| TEXAS INSTRUMENTS INCORPORATED
| Standard Linear and Logic Group
| IBIS Model of SN74LVCH245A
| OCTAL BUS TRANSCEIVERS WITH 3-STATE OUTPUTS
| This file contains package information for the following:
|  TSSOP 20-pin (PW) package as [Component] LVCH245A_PW
|  SOP 20-pin (NS) package as [Component] LVCH245A_NS
|  SOIC 20-pin (DW) package as [Component] LVCH245A_DW
|  TVSOP 20-pin (DGV) package as [Component] LVCH245A_DGV
|  SSOP 20-pin (DB) package as [Component] LVCH245A_DB
|  QFN 20-pin (RGY) package as [Component] LVCH245A_RGY
|  VFBGA 20-pin (GQN) package as [Component] LVCH245A_GQN
|  VFBGA 20-pin (ZQN) package as [Component] LVCH245A_ZQN
| This device can be powered at the following Vccs:
|  1.8 volt Vcc
|  2.5 volt Vcc
|  3.3 volt Vcc
| This file provides unique models under the [Model Selector] for each Vcc.
| For operation at a specific Vcc, select the appropriate model after each
| [Model Selector] keyword.
[IBIS Ver]   3.2
[Comment char]  |_char
[File Name]   sn74lvch245a.ibs
[File Rev]   1.2 | e_die
[Date]   November 10, 2005
[Source]   Data created from TI-SPICE simulations at TI-SLL.
[Notes]   The following is an IBIS list for the LVCH245A.
   Please contact sllibis@ti.com with questions and
   comments concerning SLL IBIS models.
   - FILE REV HISTORY
   - 1.1 Release IBIS file on 4/25/02
   - 1.2 RGY and ZQN pacakages added 11/10/05
   - Non-monotonic data in ground-clamp due to bus-hold
   - Due to the fact that the device is 5-V input/output
   tolerant, the output model has some Non-monotonic
   warnings.
[Disclaimer] Property of Texas Instruments Incorporated.  Unauthorized
   reproduction and/or distribution is strictly prohibited.
   This product is protected under copyright law.
   Created  2002, (C) Copyright  2002, Texas Instruments
   Incorporated, All Rights Reserved
   UNLESS THERE IS A SIGNED, WRITTEN AGREEMENT TO THE
   CONTRARY, TEXAS INSTRUMENTS (TI) IS PROVIDING THE IBIS
   MODELS  AND WITHOUT ANY WARRANTY, EXPRESSED OR
   IMPLIED.  TI assumes no liability for:
   1) the accuracy of the IBIS models provided to your
   company;
   2) the proper functioning of these IBIS Models in your
   design or for any resulting applications; or
   3) infringement of patents, copyrights or intellectual
   property rights resulting from your use of these IBIS
   models.
   TI provides IBIS Models as a service to our customers.
   You and your company shall not distribute, sell or give
   these models to anyone else without prior written
   permission from TI.
   TI reserves the right to make changes to our products or
   to discontinue any semiconductor product or service
   without notice, and advises our customers to obtain the
   latest version of relevant information to verify, before
   placing orders, that the information being relied on is
   current.
   Please be aware that your receipt and use of the IBIS
   information provided shall serve as acceptance of these
   terms and conditions.  If you do not accept these terms,
   you should return or destroy the IBIS models and any
   other accompanying information immediately.
| Component LVCH245A_PW 20-pin TSSOP
[Component]   LVCH245A_PW
[Manufacturer]   Texas Instruments, Inc.
[Package]
|   typ   min   max
R_pkg   4.500e-02   3.600e-02   5.700e-02
L_pkg   2.694e-09   2.290e-09   3.177e-09
C_pkg   1.560e-13   7.600e-14   2.590e-13
[Pin]   signal_name   model_name   R_pin   L_pin   C_pin
1   DIR   LVCH245A_IN   3.600e-02   3.045e-09   2.590e-13
2   A1   LVCH245A_IO   5.100e-02   3.013e-09   1.890e-13
3   A2   LVCH245A_IO   4.400e-02   2.695e-09   1.640e-13
4   A3   LVCH245A_IO   4.700e-02   2.362e-09   7.900e-14
5   A4   LVCH245A_IO   4.700e-02   2.333e-09   8.600e-14
6   A5   LVCH245A_IO   4.700e-02   2.298e-09   8.500e-14
7   A6   LVCH245A_IO   4.700e-02   2.351e-09   7.900e-14
8   A7   LVCH245A_IO   4.400e-02   2.706e-09   1.650e-13
9   A8   LVCH245A_IO   4.900e-02   2.999e-09   1.880e-13
10   GND   GND   3.900e-02   3.039e-09   2.570e-13
11   B8   LVCH245A_IO   3.800e-02   3.044e-09   2.580e-13
12   B7   LVCH245A_IO   5.700e-02   3.177e-09   1.990e-13
13   B6   LVCH245A_IO   4.400e-02   2.825e-09   1.730e-13
14   B5   LVCH245A_IO   4.700e-02   2.429e-09   8.300e-14
15   B4   LVCH245A_IO   4.900e-02   2.383e-09   9.000e-14
16   B3   LVCH245A_IO   4.900e-02   2.347e-09   8.900e-14
17   B2   LVCH245A_IO   4.700e-02   2.290e-09   7.600e-14
18   B1   LVCH245A_IO   4.500e-02   2.613e-09   1.580e-13
19   NOE   LVCH245A_IN   4.400e-02   2.883e-09   1.810e-13
20   VCC   POWER   3.900e-02   3.044e-09   2.560e-13
| Component LVCH245A_NS 20-pin SOP
[Component]   LVCH245A_NS
[Manufacturer]   Texas Instruments, Inc.
[Package]
|   typ   min   max
R_pkg   4.400e-02   2.900e-02   5.800e-02
L_pkg   3.666e-09   2.317e-09   5.115e-09
C_pkg   5.480e-13   3.160e-13   7.250e-13
[Pin]   signal_name   model_name   R_pin   L_pin   C_pin
1   DIR   LVCH245A_IN   5.800e-02   5.115e-09   7.250e-13
2   A1   LVCH245A_IO   5.300e-02   4.591e-09   7.240e-13
3   A2   LVCH245A_IO   4.900e-02   3.754e-09   5.720e-13
4   A3   LVCH245A_IO   2.900e-02   2.549e-09   3.880e-13
5   A4   LVCH245A_IO   3.100e-02   2.317e-09   3.160e-13
6   A5   LVCH245A_IO   3.100e-02   2.317e-09   3.160e-13
7   A6   LVCH245A_IO   2.900e-02   2.556e-09   3.990e-13
8   A7   LVCH245A_IO   4.900e-02   3.754e-09   5.790e-13
9   A8   LVCH245A_IO   5.300e-02   4.591e-09   7.240e-13
10   GND   GND   5.800e-02   5.115e-09   7.250e-13
11   B8   LVCH245A_IO   5.800e-02   5.115e-09   7.250e-13
12   B7   LVCH245A_IO   5.300e-02   4.591e-09   7.240e-13
13   B6   LVCH245A_IO   4.900e-02   3.754e-09   5.790e-13
14   B5   LVCH245A_IO   2.900e-02   2.557e-09   3.990e-13
15   B4   LVCH245A_IO   3.100e-02   2.317e-09   3.160e-13
16   B3   LVCH245A_IO   3.100e-02   2.317e-09   3.160e-13
17   B2   LVCH245A_IO   2.900e-02   2.557e-09   3.990e-13
18   B1   LVCH245A_IO   4.900e-02   3.754e-09   5.790e-13
19   NOE   LVCH245A_IN   5.300e-02   4.591e-09   7.240e-13
20   VCC   POWER   5.800e-02   5.115e-09   7.250e-13
| Component LVCH245A_DW 20-pin SOIC
[Component]   LVCH245A_DW
[Manufacturer]   Texas Instruments, Inc.
[Package]
|   typ   min   max
R_pkg   3.800e-02   3.300e-02   4.500e-02
L_pkg   5.012e-09   4.110e-09   6.349e-09
C_pkg   7.170e-13   5.300e-13   8.680e-13
[Pin]   signal_name   model_name   R_pin   L_pin   C_pin
1   DIR   LVCH245A_IN   4.200e-02   6.336e-09   8.650e-13
2   A1   LVCH245A_IO   4.300e-02   5.542e-09   8.670e-13
3   A2   LVCH245A_IO   3.400e-02   4.714e-09   7.320e-13
4   A3   LVCH245A_IO   3.400e-02   4.377e-09   5.910e-13
5   A4   LVCH245A_IO   3.600e-02   4.130e-09   5.330e-13
6   A5   LVCH245A_IO   3.500e-02   4.111e-09   5.300e-13
7   A6   LVCH245A_IO   3.400e-02   4.284e-09   5.830e-13
8   A7   LVCH245A_IO   3.400e-02   4.634e-09   7.260e-13
9   A8   LVCH245A_IO   4.000e-02   5.518e-09   8.650e-13
10   GND   GND   4.300e-02   6.349e-09   8.660e-13
11   B8   LVCH245A_IO   4.100e-02   6.281e-09   8.610e-13
12   B7   LVCH245A_IO   4.500e-02   5.561e-09   8.680e-13
13   B6   LVCH245A_IO   3.300e-02   4.778e-09   7.420e-13
14   B5   LVCH245A_IO   3.500e-02   4.414e-09   5.960e-13
15   B4   LVCH245A_IO   3.500e-02   4.110e-09   5.330e-13
16   B3   LVCH245A_IO   3.600e-02   4.130e-09   5.330e-13
17   B2   LVCH245A_IO   3.400e-02   4.377e-09   5.910e-13
18   B1   LVCH245A_IO   3.400e-02   4.714e-09   7.310e-13
19   NOE   LVCH245A_IN   4.300e-02   5.569e-09   8.680e-13
20   VCC   POWER   4.200e-02   6.308e-09   8.640e-13
| Component LVCH245A_DGV 20-pin TVSOP
[Component]   LVCH245A_DGV
[Manufacturer]   Texas Instruments, Inc.
[Package]
|   typ   min   max
R_pkg   4.400e-02   3.800e-02   4.800e-02
L_pkg   2.561e-09   2.236e-09   2.961e-09
C_pkg   3.420e-13   2.640e-13   4.460e-13
[Pin]   signal_name   model_name   R_pin   L_pin   C_pin
1   DIR   LVCH245A_IN   4.400e-02   2.935e-09   4.170e-13
2   A1   LVCH245A_IO   4.200e-02   2.869e-09   4.460e-13
3   A2   LVCH245A_IO   4.300e-02   2.399e-09   3.160e-13
4   A3   LVCH245A_IO   4.400e-02   2.236e-09   2.650e-13
5   A4   LVCH245A_IO   4.600e-02   2.278e-09   2.640e-13
6   A5   LVCH245A_IO   4.500e-02   2.274e-09   2.640e-13
7   A6   LVCH245A_IO   4.400e-02   2.285e-09   2.690e-13
8   A7   LVCH245A_IO   4.300e-02   2.452e-09   3.200e-13
9   A8   LVCH245A_IO   4.400e-02   2.900e-09   4.460e-13
10   GND   GND   4.400e-02   2.961e-09   4.180e-13
11   B8   LVCH245A_IO   4.500e-02   2.954e-09   4.180e-13
12   B7   LVCH245A_IO   4.200e-02   2.847e-09   4.430e-13
13   B6   LVCH245A_IO   4.500e-02   2.453e-09   3.190e-13
14   B5   LVCH245A_IO   4.500e-02   2.297e-09   2.690e-13
15   B4   LVCH245A_IO   4.800e-02   2.334e-09   2.680e-13
16   B3   LVCH245A_IO   4.800e-02   2.335e-09   2.670e-13
17   B2   LVCH245A_IO   4.600e-02   2.299e-09   2.680e-13
18   B1   LVCH245A_IO   4.600e-02   2.457e-09   3.200e-13
19   NOE   LVCH245A_IN   4.300e-02   2.848e-09   4.410e-13
20   VCC   POWER   3.800e-02   2.812e-09   4.080e-13
| Component LVCH245A_DB 20-pin SSOP
[Component]   LVCH245A_DB
[Manufacturer]   Texas Instruments, Inc.
[Package]
|   typ   min   max
R_pkg   4.000e-02   3.500e-02   5.100e-02
L_pkg   3.495e-09   3.035e-09   4.314e-09
C_pkg   4.200e-13   3.460e-13   5.020e-13
[Pin]   signal_name   model_name   R_pin   L_pin   C_pin
1   DIR   LVCH245A_IN   4.900e-02   4.310e-09   5.020e-13
2   A1   LVCH245A_IO   4.800e-02   3.903e-09   4.870e-13
3   A2   LVCH245A_IO   3.500e-02   3.189e-09   3.960e-13
4   A3   LVCH245A_IO   3.500e-02   3.036e-09   3.470e-13
5   A4   LVCH245A_IO   3.500e-02   3.035e-09   3.670e-13
6   A5   LVCH245A_IO   3.500e-02   3.035e-09   3.670e-13
7   A6   LVCH245A_IO   3.500e-02   3.036e-09   3.470e-13
8   A7   LVCH245A_IO   3.500e-02   3.189e-09   3.970e-13
9   A8   LVCH245A_IO   4.700e-02   3.899e-09   4.880e-13
10   GND   GND   5.100e-02   4.314e-09   5.000e-13
11   B8   LVCH245A_IO   5.100e-02   4.314e-09   5.000e-13
12   B7   LVCH245A_IO   4.700e-02   3.899e-09   4.880e-13
13   B6   LVCH245A_IO   3.500e-02   3.189e-09   3.970e-13
14   B5   LVCH245A_IO   3.500e-02   3.036e-09   3.460e-13
15   B4   LVCH245A_IO   3.500e-02   3.035e-09   3.670e-13
16   B3   LVCH245A_IO   3.500e-02   3.035e-09   3.670e-13
17   B2   LVCH245A_IO   3.500e-02   3.036e-09   3.460e-13
18   B1   LVCH245A_IO   3.500e-02   3.189e-09   3.970e-13
19   NOE   LVCH245A_IN   4.700e-02   3.899e-09   4.880e-13
20   VCC   POWER   5.100e-02   4.314e-09   5.020e-13
| Component LVCH245A_RGY 20-pin QFN
[Component]   LVCH245A_RGY
[Manufacturer]   Texas Instruments, Inc.
[Package]
|   typ   min   max
R_pkg   5.000e-02   4.600e-02   5.500e-02
L_pkg   1.119e-09   1.025e-09   1.227e-09
C_pkg   3.520e-13   3.440e-13   3.630e-13
[Pin]   signal_name   model_name   R_pin   L_pin   C_pin
1   DIR   LVCH245A_IN   5.200e-02   1.167e-09   3.600e-13
2   A1   LVCH245A_IO   4.700e-02   1.049e-09   3.440e-13
3   A2   LVCH245A_IO   4.700e-02   1.055e-09   3.450e-13
4   A3   LVCH245A_IO   5.000e-02   1.119e-09   3.500e-13
5   A4   LVCH245A_IO   5.500e-02   1.227e-09   3.600e-13
6   A5   LVCH245A_IO   5.200e-02   1.167e-09   3.550e-13
7   A6   LVCH245A_IO   4.900e-02   1.087e-09   3.480e-13
8   A7   LVCH245A_IO   4.700e-02   1.054e-09   3.460e-13
9   A8   LVCH245A_IO   4.900e-02   1.091e-09   3.490e-13
10   GND   GND   5.300e-02   1.184e-09   3.620e-13
11   B8   LVCH245A_IO   5.300e-02   1.181e-09   3.600e-13
12   B7   LVCH245A_IO   5.000e-02   1.108e-09   3.490e-13
13   B6   LVCH245A_IO   4.800e-02   1.075e-09   3.470e-13
14   B5   LVCH245A_IO   5.000e-02   1.107e-09   3.490e-13
15   B4   LVCH245A_IO   5.400e-02   1.200e-09   3.620e-13
16   B3   LVCH245A_IO   5.100e-02   1.141e-09   3.570e-13
17   B2   LVCH245A_IO   4.700e-02   1.043e-09   3.440e-13
18   B1   LVCH245A_IO   4.600e-02   1.025e-09   3.440e-13
19   NOE   LVCH245A_IN   4.900e-02   1.090e-09   3.490e-13
20   VCC   POWER   5.400e-02   1.204e-09   3.630e-13
| Component LVCH245A_GQN 20-pin VFBGA
[Component]   LVCH245A_GQN
[Manufacturer] Texas Instruments, Inc.
[Package]
|   typ   min   max
R_pkg   4.300e-02   3.300e-02   6.100e-02
L_pkg   1.317e-09   8.960e-10   2.088e-09
C_pkg   1.130e-13   6.400e-14   1.900e-13
[Pin]   signal_name   model_name   R_pin   L_pin   C_pin
A2   DIR   LVCH245A_IN   3.800e-02   1.199e-09   1.210e-13
A1   A1   LVCH245A_IO   4.000e-02   1.067e-09   1.020e-13
B3   A2   LVCH245A_IO   6.100e-02   1.999e-09   1.900e-13
B1   A3   LVCH245A_IO   3.300e-02   9.630e-10   7.100e-14
C2   A4   LVCH245A_IO   4.900e-02   1.523e-09   1.230e-13
C1   A5   LVCH245A_IO   3.300e-02   8.960e-10   6.400e-14
D3   A6   LVCH245A_IO   6.100e-02   1.899e-09   1.640e-13
D1   A7   LVCH245A_IO   3.300e-02   8.980e-10   6.700e-14
E2   A8   LVCH245A_IO   4.900e-02   1.514e-09   1.280e-13
E1   GND   GND   3.600e-02   1.006e-09   9.400e-14
E3   B8   LVCH245A_IO   4.900e-02   1.683e-09   1.460e-13
E4   B7   LVCH245A_IO   3.300e-02   1.121e-09   8.900e-14
D2   B6   LVCH245A_IO   6.100e-02   2.088e-09   1.730e-13
D4   B5   LVCH245A_IO   3.300e-02   1.027e-09   7.100e-14
C3   B4   LVCH245A_IO   4.900e-02   1.558e-09   1.240e-13
C4   B3   LVCH245A_IO   3.300e-02   9.280e-10   6.700e-14
B2   B2   LVCH245A_IO   6.100e-02   1.921e-09   1.770e-13
B4   B1   LVCH245A_IO   3.300e-02   9.010e-10   7.700e-14
A4   NOE   LVCH245A_IN   3.700e-02   9.900e-10   9.800e-14
A3   VCC   POWER   3.500e-02   1.168e-09   1.190e-13
| Component LVCH245A_ZQN 20-pin VFBGA
[Component]   LVCH245A_ZQN
[Manufacturer] Texas Instruments, Inc.
[Package]
|   typ   min   max
R_pkg   4.300e-02   3.300e-02   6.100e-02
L_pkg   1.317e-09   8.960e-10   2.088e-09
C_pkg   1.130e-13   6.400e-14   1.900e-13
[Pin]   signal_name   model_name   R_pin   L_pin   C_pin
A2   DIR   LVCH245A_IN   3.800e-02   1.199e-09   1.210e-13
A1   A1   LVCH245A_IO   4.000e-02   1.067e-09   1.020e-13
B3   A2   LVCH245A_IO   6.100e-02   1.999e-09   1.900e-13
B1   A3   LVCH245A_IO   3.300e-02   9.630e-10   7.100e-14
C2   A4   LVCH245A_IO   4.900e-02   1.523e-09   1.230e-13
C1   A5   LVCH245A_IO   3.300e-02   8.960e-10   6.400e-14
D3   A6   LVCH245A_IO   6.100e-02   1.899e-09   1.640e-13
D1   A7   LVCH245A_IO   3.300e-02   8.980e-10   6.700e-14
E2   A8   LVCH245A_IO   4.900e-02   1.514e-09   1.280e-13
E1   GND   GND   3.600e-02   1.006e-09   9.400e-14
E3   B8   LVCH245A_IO   4.900e-02   1.683e-09   1.460e-13
E4   B7   LVCH245A_IO   3.300e-02   1.121e-09   8.900e-14
D2   B6   LVCH245A_IO   6.100e-02   2.088e-09   1.730e-13
D4   B5   LVCH245A_IO   3.300e-02   1.027e-09   7.100e-14
C3   B4   LVCH245A_IO   4.900e-02   1.558e-09   1.240e-13
C4   B3   LVCH245A_IO   3.300e-02   9.280e-10   6.700e-14
B2   B2   LVCH245A_IO   6.100e-02   1.921e-09   1.770e-13
B4   B1   LVCH245A_IO   3.300e-02   9.010e-10   7.700e-14
A4   NOE   LVCH245A_IN   3.700e-02   9.900e-10   9.800e-14
A3   VCC   POWER   3.500e-02   1.168e-09   1.190e-13
| Model LVCH245A_IN
[Model Selector]   LVCH245A_IN
LVCH245A_IN_18   1.8 volt Vcc
LVCH245A_IN_25   2.5 volt Vcc
LVCH245A_IN_33   3.3 volt Vcc
| Model LVCH245A_IO
[Model Selector]   LVCH245A_IO
LVCH245A_IO_18   1.8 volt Vcc
LVCH245A_IO_25   2.5 volt Vcc
LVCH245A_IO_33   3.3 volt Vcc
| Models and submodels in the file (6): LVCH245A_IN_18 (Input), LVCH245A_IN_25 (Input), LVCH245A_IN_33 (Input), LVCH245A_IO_18 (I/O), LVCH245A_IO_25 (I/O), LVCH245A_IO_33 (I/O)
